{attribute 'pack_mode' := '8'}
TYPE ST_EL5131_CamData :
STRUCT
	bVaild				:	BOOL;// Mutil_Cycle 时有用，Single_Cylce 时忽略该变量
	bOutputState		:	BOOL;
	bBackward			:	BOOL;// =1反向，=0正向 备用
	{attribute 'hide'}
	reserve_b4			:	BOOL;
	nDuration			:	UDINT;
	rPos				:	LREAL;
END_STRUCT
END_TYPE
